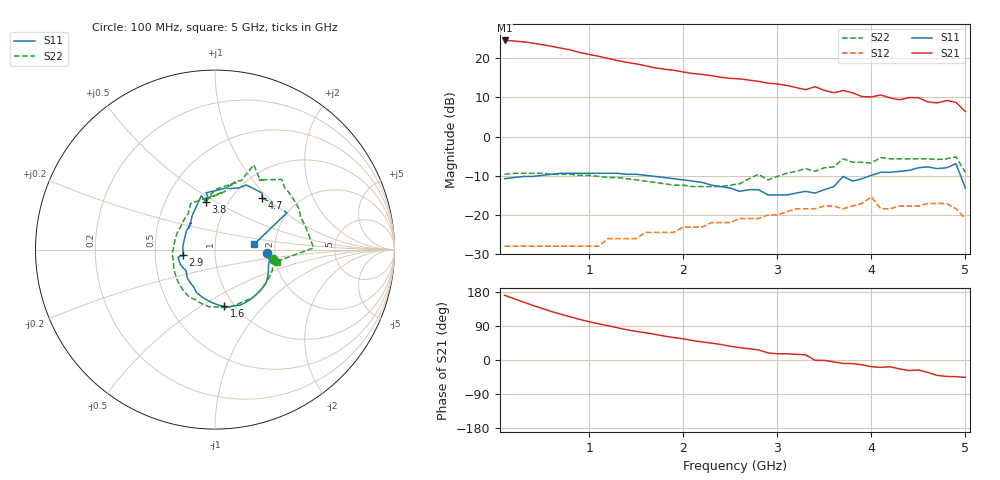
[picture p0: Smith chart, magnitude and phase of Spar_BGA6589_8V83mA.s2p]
!BGA6589
!Scattering parameters
!Is=83mA Vs=8V
!Pd=-30dBm
!Z0=50 Ohm
!Tamb 25C
#  MHz  S  MA  R 50
! Freq  S11  S21  S12  S22  :
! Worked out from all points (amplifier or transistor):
!   50 points, 100 MHz to 5 GHz, reference 50 ohm
!   highest |S21| = 24.5 dB at 100 MHz (marker M1)
!   |S21| within 3 dB of that: start of sweep to 888.9 MHz
!   unconditionally stable (mu >= 1): start of sweep to end of sweep
!   at 900 MHz: K = 1.11, MAG = 22.7 dB, |S12| = -28.0 dB
!   at 2.6 GHz: K = 1.15, MAG = 15.4 dB, |S12| = -20.9 dB
!   at 5 GHz: K = 2.26, MAG = 7.3 dB, |S12| = -20.9 dB
!   S11 on the Smith chart (normalised r, x): 100 MHz: 1.81, -0.07; 1.6 GHz: 0.90, -0.63; 2.9 GHz: 0.70, -0.04; 3.8 GHz: 0.79, +0.45; 4.7 GHz: 1.36, +0.92; 5 GHz: 1.55, +0.10
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100  0.29 -3.5  16.79 170.8  0.04 1.4  0.33 -9.3
300  0.31 -11.3  16.1 152.9  0.04 3.7  0.34 -31.2
500  0.32 -21.6  14.83 135.8  0.04 6.8  0.34 -51.7
700  0.34 -32.8  13.41 120.6  0.04 11.0  0.33 -70.8
800  0.34 -38.5  12.69 113.8  0.04 13.7  0.33 -79.6
1000  0.34 -49.9  11.12 101.0  0.04 18.0  0.32 -96.0
1400  0.33 -71.0  8.82 79.8  0.05 24.6  0.29 -126.3
1600  0.32 -81.0  7.98 71.8  0.06 27.6  0.27 -141.2
1800  0.3 -91.1  7.22 63.0  0.06 28.1  0.25 -157.0
2600  0.2 -143.6  5.43 32.7  0.09 24.3  0.25 126.7
2800  0.21 -168.4  5.05 26.7  0.09 24.1  0.33 80.0
2900  0.18 -170.2  4.79 18.7  0.1 19.9  0.28 102.8
3300  0.2 131.6  3.95 13.5  0.12 18.8  0.39 72.7
3400  0.19 140.8  4.32 -0.7  0.12 7.4  0.36 78.2
3600  0.23 123.2  3.62 -5.2  0.13 6.9  0.41 69.2
3800  0.27 100.9  3.62 -9.5  0.13 2.3  0.47 58.5
3900  0.29 97.1  3.23 -12.7  0.14 0.5  0.47 55.5
4200  0.35 75.9  3.11 -17.9  0.12 -10.3  0.52 41.9
4500  0.4 64.2  3.13 -26.3  0.13 -11.7  0.52 30.2
4700  0.39 47.3  2.68 -40.7  0.14 -16.3  0.51 20.7
4900  0.45 27.1  2.73 -44.2  0.12 -23.7  0.55 1.0
5000  0.22 7.8  2.08 -45.7  0.09 7.3  0.35 -10.9
